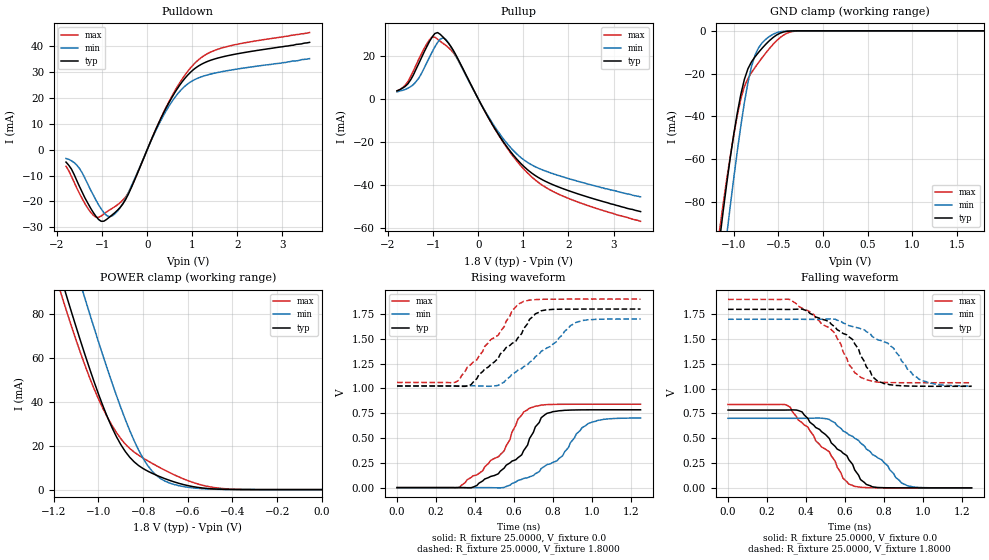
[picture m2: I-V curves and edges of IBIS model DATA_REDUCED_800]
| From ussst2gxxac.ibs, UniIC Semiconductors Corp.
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|   Model DATA_REDUCED_800
[Model]  DATA_REDUCED_800
Model_type I/O
Polarity   Non-Inverting
Enable   Active-High
Vinl =   0.70000000V
Vinh =   1.10000000V
Vmeas =   0.90000000V
Rref =   25.00000000
Vref =   0.90000000V
C_comp   2.5240pF   2.5060pF   2.5510pF
[Temperature Range]   25.0000   95.0000   0.0
[Voltage Range]   1.8000V   1.7000V   1.9000V
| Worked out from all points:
|   slope of the pulldown table from 0 to 0.27 V, typ, clamps not added: 24.9 ohm
|   slope of the pullup table from 0 to 0.27 V, typ, clamps not added: 26.2 ohm
|   GND clamp passes 1 mA (typ) near -0.47 V on its own axis
|   POWER clamp passes 1 mA (typ) near -0.55 V on its own axis
|   rising waveform, R_fixture 25.0000, V_fixture 0.0: 20-80 % time 190ps typ, 221ps min, 179ps max; typ from 0 V to 0.784 V
|   rising waveform, R_fixture 25.0000, V_fixture 1.8000: 20-80 % time 223ps typ, 251ps min, 209ps max; typ from 1.02 V to 1.8 V
|   falling waveform, R_fixture 25.0000, V_fixture 0.0: 20-80 % time 217ps typ, 248ps min, 205ps max; typ from 0.784 V to 0 V
|   falling waveform, R_fixture 25.0000, V_fixture 1.8000: 20-80 % time 195ps typ, 222ps min, 183ps max; typ from 1.8 V to 1.02 V
[Pulldown]
|Voltage   I(typ)   I(min)   I(max)
-1.8V     -4.8mA     -3.4mA     -6.4mA
-1.5V     -14.3mA    -7.3mA     -17mA
-1.26V    -22.5mA    -15.4mA    -24.1mA
-1.14V    -25.73mA   -19.4mA    -26.15mA
-960mV    -27.7mA    -24.4mA    -24.93mA
-720mV    -24.45mA   -24.93mA   -22.1mA
-420mV    -17.33mA   -16.79mA   -16.77mA
420mV     16.17mA    15.06mA    16.48mA
720mV     24.99mA    22.57mA    25.9mA
1.02V     30.95mA    26.87mA    32.88mA
1.68V     36.02mA    30.33mA    39.55mA
3.6V      41.6mA     35.3mA     45.4mA
[Pullup]
|Voltage   I(typ)   I(min)   I(max)
-1.8V     3.7mA      3.2mA      3.6mA
-1.56V    6.9mA      4.9mA      7.9mA
-1.38V    13.6mA     7.9mA      15.5mA
-1.08V    26.53mA    19.24mA    27.32mA
-900mV    30.65mA    26.1mA     27.55mA
-780mV    28.58mA    28.2mA     25.65mA
-660mV    25.76mA    25.92mA    23.72mA
-420mV    17.3mA     16.82mA    17.01mA
360mV     -13.47mA   -12.68mA   -13.61mA
1.08V     -32.59mA   -29.26mA   -34.06mA
1.86V     -41.45mA   -36.02mA   -44.87mA
3.6V      -52.2mA    -45.4mA    -56.7mA
[GND_clamp]
|Voltage   I(typ)   I(min)   I(max)
-1.8V     -341.4mA   -368.9mA   -332.4mA
-1.16V    -98.84mA   -124.9mA   -94.02mA
-1.12V    -85.23mA   -110.5mA   -81.66mA
-1.08V    -72.2mA    -96.41mA   -70.06mA
-1.04V    -59.93mA   -82.62mA   -59.18mA
-920mV    -29.77mA   -44.48mA   -31.9mA
-880mV    -22.69mA   -33.57mA   -26.06mA
-800mV    -14.49mA   -16.62mA   -19.53mA
-720mV    -10.02mA   -7.817mA   -14.76mA
-560mV    -3.159mA   -1.628mA   -6.393mA
-280mV    -8.14uA    -3.578uA   -70uA
1.8V      7.234nA    32.16nA    61.22nA
[POWER_clamp]
|Voltage   I(typ)   I(min)   I(max)
-1.8V     325.1mA    352.4mA    316.2mA
-1.16V    94.14mA    121mA      86.98mA
-1.14V    87.41mA    114.1mA    80.57mA
-1.06V    61.46mA    87.09mA    56.62mA
-980mV    38.21mA    61.22mA    37.03mA
-900mV    20.56mA    37.47mA    23.27mA
-820mV    10.96mA    18mA       15.69mA
-780mV    8.467mA    11.05mA    13.18mA
-740mV    6.55mA     6.435mA    10.88mA
-640mV    2.87mA     1.791mA    5.795mA
-480mV    290.4uA    171.3uA    911.2uA
0V        7.234nA    10.13nA    70.66nA
[Ramp]
| variable   typ   min   max
dV/dt_r  0.4706/0.1900n   0.4209/0.2336n   0.5044/0.1772n
dV/dt_f  0.4656/0.1909n   0.4044/0.2349n   0.5040/0.1786n
R_load = 25.0000
[Rising Waveform]
R_fixture= 25.0000
V_fixture= 0.0
V_fixture_min= 0.0
V_fixture_max= 0.0
|time   V(typ)   V(min)   V(max)
0s        0V         0V         0V
320ps     220.1uV    -3.424uV   2.441mV
410ps     21.62mV    136.8uV    128.6mV
550ps     196.4mV    1.666mV    371.1mV
620ps     300.1mV    71.36mV    687.9mV
680ps     494mV      108.4mV    800.8mV
770ps     748.9mV    231.5mV    836.8mV
850ps     777.2mV    321.2mV    839.9mV
980ps     784mV      645mV      840.6mV
1.25ns    784.4mV    701.5mV    840.6mV
[Rising Waveform]
R_fixture= 25.0000
V_fixture= 1.8000
V_fixture_min= 1.7000
V_fixture_max= 1.9000
|time   V(typ)   V(min)   V(max)
0s        1.024V     1.026V     1.06V
320ps     1.022V     1.026V     1.084V
380ps     1.037V     1.026V     1.242V
480ps     1.239V     1.022V     1.49V
520ps     1.305V     1.031V     1.537V
590ps     1.453V     1.143V     1.783V
650ps     1.602V     1.219V     1.878V
740ps     1.782V     1.374V     1.898V
920ps     1.799V     1.667V     1.9V
1.25ns    1.8V       1.7V       1.9V
[Falling Waveform]
R_fixture= 25.0000
V_fixture= 0.0
V_fixture_min= 0.0
V_fixture_max= 0.0
|time   V(typ)   V(min)   V(max)
0s        784.4mV    701.5mV    840.6mV
320ps     785.4mV    701.4mV    812.3mV
380ps     765.8mV    701.3mV    658mV
520ps     497.3mV    689.7mV    363.8mV
590ps     350.6mV    574.1mV    97.38mV
650ps     181mV      500.1mV    15.12mV
680ps     83.81mV    453mV      6.006mV
740ps     11mV       337.9mV    801.6uV
920ps     36.75uV    21.57mV    2.584uV
1.25ns    0V         0V         0V
[Falling Waveform]
R_fixture= 25.0000
V_fixture= 1.8000
V_fixture_min= 1.7000
V_fixture_max= 1.9000
|time   V(typ)   V(min)   V(max)
0s        1.8V       1.7V       1.9V
320ps     1.799V     1.7V       1.899V
550ps     1.621V     1.7V       1.556V
610ps     1.543V     1.648V     1.304V
650ps     1.453V     1.619V     1.162V
710ps     1.22V      1.575V     1.089V
770ps     1.073V     1.492V     1.066V
850ps     1.036V     1.408V     1.061V
980ps     1.025V     1.096V     1.06V
1.25ns    1.024V     1.026V     1.06V
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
